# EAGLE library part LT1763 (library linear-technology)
500mA, Low Noise, LDO Micropower Regulators Source: http://cds.linear.com/docs/Datasheet/1763ff.pdf
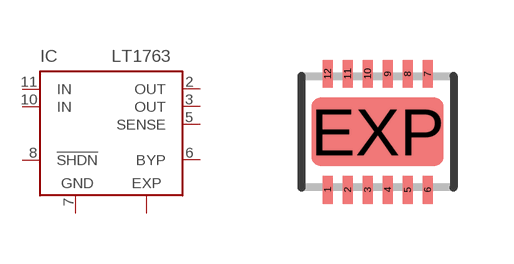
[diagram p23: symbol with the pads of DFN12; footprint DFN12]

Designator prefix IC

## LT1763CDE (MPN: LT1763CDE; OC_FARNELL: 1273613; OC_NEWARK: 57M6014), LT1763CDE-1.5 (MPN: LT1763CDE-1.5; OC_FARNELL: unknown; OC_NEWARK: 57M6015), LT1763CDE-1.8 (MPN: LT1763CDE-1.8; OC_FARNELL: unknown; OC_NEWARK: 57M6019), LT1763CDE-2.5 (MPN: LT1763CDE-2.5; OC_FARNELL: unknown; OC_NEWARK: 57M6023), LT1763CDE-3 (MPN: LT1763CDE-3; OC_FARNELL: unknown; OC_NEWARK: 57M6027), LT1763CDE-3.3 (MPN: LT1763CDE-3.3; OC_FARNELL: unknown; OC_NEWARK: 57M6028), LT1763CDE-5 (MPN: LT1763CDE-5; OC_FARNELL: 1556468; OC_NEWARK: 57M6035), LT1763IDE (MPN: LT1763IDE#PBF; OC_FARNELL: 1839216; OC_NEWARK: 51R1532), LT1763IDE-1.5 (MPN: LT1763IDE-1.5#PBF; OC_FARNELL: 1783317; OC_NEWARK: 51R1526), LT1763IDE-1.8 (MPN: LT1763IDE-1.8#PBF; OC_FARNELL: 1783318; OC_NEWARK: 51R1527), LT1763IDE-2.5 (MPN: LT1763IDE-2.5#PBF; OC_FARNELL: 1783319; OC_NEWARK: 51R1528), LT1763IDE-3 (MPN: LT1763IDE-3#PBF; OC_FARNELL: 1839220; OC_NEWARK: 51R1530), LT1763IDE-3.3 (MPN: LT1763IDE-3.3#PBF; OC_FARNELL: 1783320; OC_NEWARK: 51R1529), LT1763IDE-5 (MPN: LT1763IDE-5#PBF; OC_FARNELL: 1839222; OC_NEWARK: 51R1531)  [DFN12]
2  OUT  pas
3  OUT  pas
5  SENSE  in
6  BYP  in
7  GND  pwr
8  !SHDN  in
10  IN  in
11  IN  in
EXP  EXP  pwr

## Footprint DFN12 (pad centres in mm)
DE/UE Package 12-Lead Plastic DFN (4mm × 3mm) Source: http://cds.linear.com/docs/Datasheet/1763ff.pdf
smd 0.25 x 0.7: 1 -1.25,-1.45; 2 -0.75,-1.45; 3 -0.25,-1.45; 4 0.25,-1.45; 5 0.75,-1.45; 6 1.25,-1.45; 7 1.25,1.45; 8 0.75,1.45; 9 0.25,1.45; 10 -0.25,1.45; 11 -0.75,1.45; 12 -1.25,1.45
smd 3.3 x 1.7: EXP 0,0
